(* Logix 5000 AddOnInstructionDefinition export; software revision 16.04 *)

ADD_ON_INSTRUCTION AMCI_ANG1E_Clear_driver_fault   (* revision 1.1, vendor AMCI *)
// Revision note:
// Version 1.1 added the slot_axis number and the input parameters can now be tags or discrete values.
VAR_INPUT
   slot_axis_number : INT; {required}
END_VAR
VAR_IN_OUT
   AMCI_ANG1E_output_data : INT[10]; {required}
END_VAR
VAR
   command_data_block : INT[10];
        [0]   // Command Bits MSW
        [1]   // Command Bits LSW
        [2]   // Upper Target Position
        [3]   // Lower Target Position
        [4]   // Upper Programmed Speed
        [5]   // Lower Programmed Speed
   index : INT;
END_VAR

ROUTINE Logic   (* ladder *)
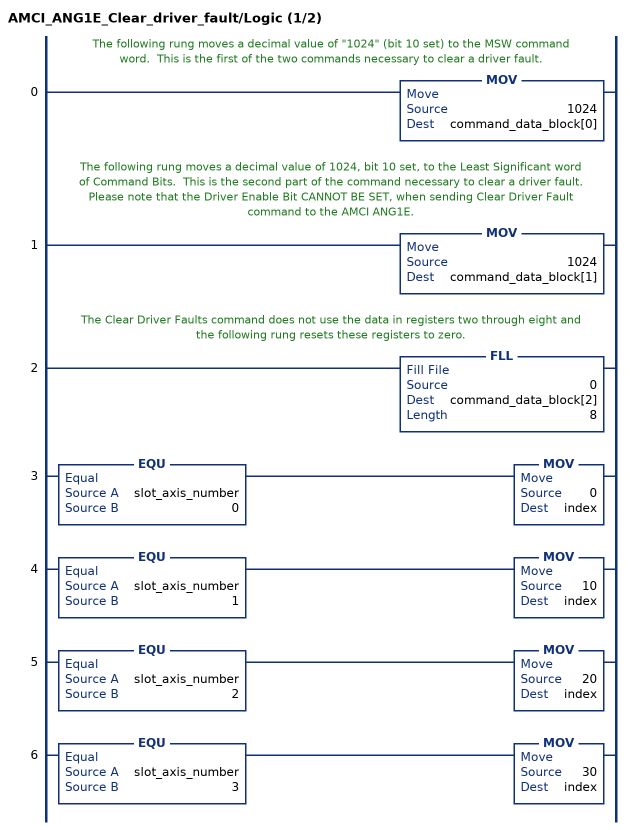
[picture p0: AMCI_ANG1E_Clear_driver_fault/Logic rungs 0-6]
   // The following rung moves a decimal value of "1024" (bit 10 set) to the MSW command word.  This is the first of the two commands necessary to clear a driver fault.
   0: MOV(1024,command_data_block[0]);
   // The following rung moves a decimal value of 1024, bit 10 set, to the Least Significant word of Command Bits.  This is the second part of the command necessary to clear a driver fault.
   // Please note that the Driver Enable Bit CANNOT BE SET, when sending Clear Driver Fault command to the AMCI ANG1E.
   1: MOV(1024,command_data_block[1]);
   // The Clear Driver Faults command does not use the data in registers two through eight and the following rung resets these registers to zero.
   2: FLL(0,command_data_block[2],8);
   3: EQU(slot_axis_number,0)MOV(0,index);
   4: EQU(slot_axis_number,1)MOV(10,index);
   5: EQU(slot_axis_number,2)MOV(20,index);
   6: EQU(slot_axis_number,3)MOV(30,index);
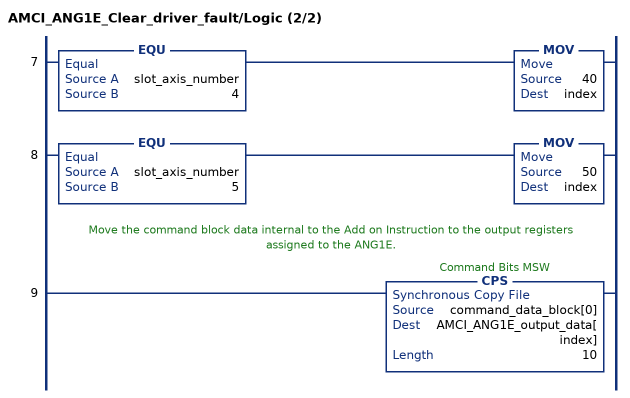
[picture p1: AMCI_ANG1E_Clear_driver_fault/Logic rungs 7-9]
   7: EQU(slot_axis_number,4)MOV(40,index);
   8: EQU(slot_axis_number,5)MOV(50,index);
   // Move the command block data internal to the Add on Instruction to the output registers assigned to the ANG1E.
   9: CPS(command_data_block[0],AMCI_ANG1E_output_data[index],10);
END_ROUTINE
END_ADD_ON_INSTRUCTION
